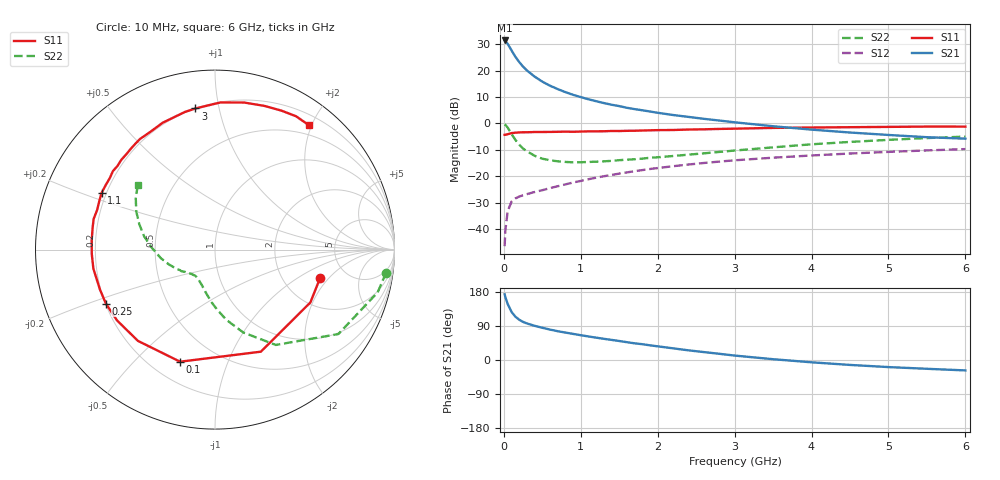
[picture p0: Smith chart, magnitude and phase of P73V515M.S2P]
! SIEMENS Small Signal Semiconductors
! BFP196
! Si NPN RF Bipolar Junction Transistor in SOT143
! VCE = 3.5 V  IC = 15 mA
! Common Emitter S-Parameters:  May  1996
# GHz  S  MA  R  50
!  f  S11  S21  S12  S22
! GHz  MAG  ANG  MAG  ANG  MAG  ANG  MAG  ANG
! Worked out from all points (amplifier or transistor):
!   36 points, 10 MHz to 6 GHz, reference 50 ohm
!   highest |S21| = 31.4 dB at 10 MHz (marker M1)
!   |S21| within 3 dB of that: start of sweep to 84.57 MHz
!   unconditionally stable (mu >= 1): 769.2 MHz to 3.346 GHz
!   at 250 MHz: K = 0.51, MSG = 24.4 dB, |S12| = -27.3 dB
!   at 1.4 GHz: K = 1.12, MAG = 11.2 dB, |S12| = -19.6 dB
!   at 6 GHz: K = 0.96, MSG = 2.0 dB, |S12| = -9.8 dB
!   S11 on the Smith chart (normalised r, x): 10 MHz: 3.21, -1.61; 100 MHz: 0.31, -0.69; 250 MHz: 0.20, -0.22; 1.1 GHz: 0.18, +0.23; 3 GHz: 0.20, +0.85; 6 GHz: 0.35, +1.95
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0.01  0.6066 -15.1  37.33 173.5  0.0047 85.5  0.9617 -7.7
0.02  0.6076 -29.0  36.07 165.6  0.0094 78.2  0.9373 -14.7
0.05  0.6235 -65.8  32.19 147.8  0.0217 62.4  0.833 -34.4
0.1  0.6542 -107.3  24.2 126.9  0.0328 48.0  0.6299 -57.5
0.15  0.6656 -130.2  18.29 114.3  0.0378 41.2  0.4876 -71.2
0.2  0.6736 -144.2  14.56 106.3  0.041 38.2  0.3958 -80.9
0.25  0.6782 -153.7  11.89 100.5  0.0434 37.4  0.3333 -88.1
0.3  0.6785 -160.8  10.08 96.5  0.0456 37.8  0.2957 -93.5
0.4  0.6859 -171.1  7.71 90.2  0.05 39.4  0.2429 -102.5
0.5  0.6869 -177.9  6.185 85.0  0.0541 41.6  0.214 -109.4
0.6  0.6888 175.7  5.181 80.3  0.0592 43.7  0.1998 -114.5
0.7  0.6925 170.0  4.468 76.0  0.0643 45.4  0.1909 -118.6
0.9  0.6927 161.4  3.48 68.9  0.0757 47.7  0.1826 -125.6
1.1  0.7064 153.5  2.865 62.1  0.0874 48.9  0.1857 -130.8
1.3  0.7088 145.7  2.429 55.9  0.0995 48.9  0.1908 -135.4
1.6  0.7229 136.2  1.975 47.0  0.1177 48.0  0.205 -141.4
2.2  0.7489 118.5  1.441 30.8  0.1541 43.5  0.2407 -153.4
3  0.7938 97.9  1.048 11.7  0.1995 34.9  0.3055 -171.0
3.5  0.8203 87.9  0.883 2.1  0.2237 29.0  0.3512 178.5
4.5  0.8465 71.1  0.671 -13.0  0.2683 17.9  0.4451 161.4
5.5  0.8694 58.7  0.547 -23.2  0.3074 7.0  0.527 146.9
6  0.8683 53.1  0.513 -27.5  0.3254 1.0  0.5613 140.0
